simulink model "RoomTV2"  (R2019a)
settings: Solver=ode15s  StartTime=0.0  StopTime=tend  RelTol=1e-3
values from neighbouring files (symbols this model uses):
  ACmax = 4.5    [mainV3.m]    (also in mainV3_SRC.m)
  ACmin = 0    [mainV3.m]    (also in mainV3_SRC.m)
  EHmax = 4    [mainV3.m]    (also in mainV3_SRC.m)
  EHmin = 0    [mainV3.m]    (also in mainV3_SRC.m)
  HWmax = 3    [mainV3.m]    (also in mainV3_SRC.m)
  HWmin = 0    [mainV3.m]    (also in mainV3_SRC.m)
  Kc_ac = tau_ac/(K_ac*(tauc_ac+theta_ac))    (= -1.23666666667)    [RoomTuning.m]
  Kc_eh = tau_eh/(K_eh*(tauc_eh+theta_eh))    (= 1.23666666667)    [RoomTuning.m]
  Kc_hw = tau_hw/(K_hw*(tauc_hw+theta_hw))    (= 3.13641025641)    [RoomTuning.m]
  KI_ac = Kc_ac/tauI_ac    [RoomTuning.m]
  KI_eh = Kc_eh/tauI_eh    [RoomTuning.m]
  KI_hw = Kc_hw/tauI_hw    [RoomTuning.m]
  m_in0 = 0.4    [mainOL.m]    (also in mainV3.m; mainV3_SRC.m)
  p = [m,Cp, Ufl, Afl, mfl, Cpfl]'    [mainOL.m]    (also in mainV3.m; mainV3_SRC.m)
  par_ac = [p_ac, m_in0, Cp, kT]'    [mainV3.m]    (also in mainV3_SRC.m)
  par_el = [p_el, m_in0, Cp, kT]'    [mainV3.m]    (also in mainV3_SRC.m)
  par_hw = [p_hw, m_in0, Cp, kT]'    [mainV3.m]    (also in mainV3_SRC.m)
  par_J = [p_el, p_hw, p_ac, m_in0, kv, kT]'    [mainV3.m]    (also in mainV3_SRC.m)
  QAC0 = 0    [mainOL.m]    (also in mainV3.m; mainV3_SRC.m)
  QH10 = 0    [mainOL.m]    (also in mainV3.m; mainV3_SRC.m)
  QH20 = 0    [mainOL.m]    (also in mainV3.m; mainV3_SRC.m)
  Tdes0 = T0    (= 21)    [mainV3.m]    (also in mainV3_SRC.m)
  x0 = [T0; Tfl0]    [mainOL.m]    (also in mainV3.m; mainV3_SRC.m; col_obj.m = 0.5*ones(1,82)'; Simulate1Col.m = x)
undefined symbols (not defined in the file or in its folder): objRoom, Room, spQac, spQel, spQhw
libraries: simulink x3

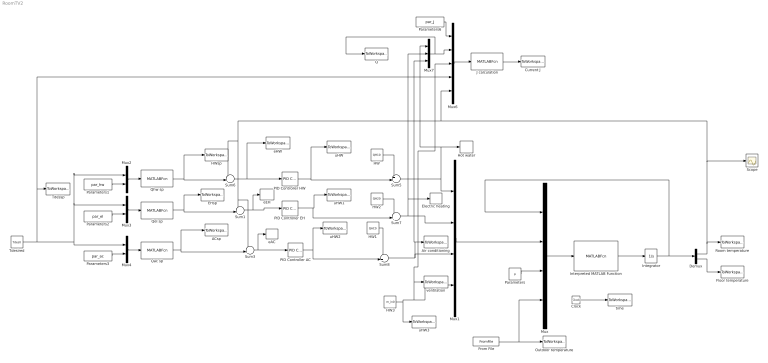
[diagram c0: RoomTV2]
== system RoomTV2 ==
  ACsp : ToWorkspace  VariableName=ACsp  SampleTime=-1
  Air conditioning : ToWorkspace  VariableName=QAC  SampleTime=-1
  Clock : Clock
  Current J : ToWorkspace  VariableName=Jactual  SampleTime=-1
  Demux : Demux  Outputs=2
  EHsp : ToWorkspace  VariableName=EHsp  SampleTime=-1
  Electric heating : ToWorkspace  VariableName=QH2  SampleTime=-1
  Floor temperature : ToWorkspace  VariableName=Tfl  SampleTime=-1
  From File : FromFile  FileName=Tambient.mat  OutDataTypeStr=double  SampleTime=0
  HW : Constant  Value=QH10
  HW1 : Constant  Value=QAC0
  HW2 : Constant  Value=QH20
  HW3 : Constant  Value=m_in0
  HWsp : ToWorkspace  VariableName=HWsp  SampleTime=-1
  Hot water : ToWorkspace  VariableName=QH1  SampleTime=-1
  Integrator : Integrator  InitialCondition=x0'
  Interpreted MATLAB Function : MATLABFcn  MATLABFcn=Room(u)  OutputDimensions=2  Output1D=off
  J calculation : MATLABFcn  MATLABFcn=objRoom(u)  OutputDimensions=1  Output1D=off
  Mux : Mux
  Mux1 : Mux
  Mux2 : Mux  Inputs=2
  Mux3 : Mux  Inputs=2
  Mux4 : Mux  Inputs=2
  Mux6 : Mux  Inputs=5
  Mux7 : Mux  Inputs=3
  Outdoor temperature : ToWorkspace  VariableName=Tin  SampleTime=-1
  PID Controller AC : simulink/Continuous/PID Controller  Controller=PI  Form=Parallel  TimeDomain=Continuous-time  SampleTime=-1  IntegratorMethod=Forward Euler  FilterMethod=Forward Euler  ControllerParametersSource=internal  P=Kc_ac  I=KI_ac  D=0  UseFilter=on  N=100  TunerSelectOption=Transfer Function Based (PID Tuner App)  InitialConditionSource=internal  InitialConditionForIntegrator=0  InitialConditionForFilter=0  DifferentiatorICPrevScaledInput=0  ExternalReset=none  TrackingMode=off  Kt=1  LimitOutput=on  UpperSaturationLimit=ACmax  LowerSaturationLimit=ACmin  LinearizeAsGain=on  AntiWindupMode=back-calculation  Kb=1  POutMin=[]  POutMax=[]  IOutMin=[]  IOutMax=[]  DOutMin=[]  DOutMax=[]  NOutMin=[]  NOutMax=[]  SumOutMin=[]  SumOutMax=[]  SaturationOutMin=[]  SaturationOutMax=[]  PParamMin=[]  PParamMax=[]  IParamMin=[]  IParamMax=[]  DParamMin=[]  DParamMax=[]  NParamMin=[]  NParamMax=[]  KbParamMin=[]  KbParamMax=[]  KtParamMin=[]  KtParamMax=[]  KbOutMin=[]  KbOutMax=[]  KtOutMin=[]  KtOutMax=[]  IntegratorOutMin=[]  IntegratorOutMax=[]  FilterOutMin=[]  FilterOutMax=[]  SumI1OutMin=[]  SumI1OutMax=[]  SumI2OutMin=[]  SumI2OutMax=[]  SumI3OutMin=[]  SumI3OutMax=[]  SumI4OutMin=[]  SumI4OutMax=[]  SumDOutMin=[]  SumDOutMax=[]  DifferentiatorOutMin=[]  DifferentiatorOutMax=[]  FilterDiffOutCoefMin=[]  FilterDiffOutCoefMax=[]  ReciprocalOutMin=[]  ReciprocalOutMax=[]  SumDenOutMin=[]  SumDenOutMax=[]  SumNumOutMin=[]  SumNumOutMax=[]  DivideOutMin=[]  DivideOutMax=[]  IntegratorContinuousStateAttributes=''  IntegratorStateMustResolveToSignalObject=off  IntegratorRTWStateStorageClass=Auto  FilterContinuousStateAttributes=''  FilterStateMustResolveToSignalObject=off  FilterRTWStateStorageClass=Auto  ParallelPVariant=InternalParameters  IdealPVariant=Disabled  IVariant=InternalParameters  DVariant=Disabled  IntegratorVariant=Continuous  SatVariant=Enabled  AWVariant=BackCalculation  PCopyVariant=Disabled  TRVariant=Disabled  FdbkBlocksVariant=Forward  IdealPFdbkVariant=Disabled  SatFdbkVariant=Disabled  DerivativeFilterVariant=Disabled  NVariant=Disabled  NCopyVariant=Disabled_SignalSpec  FilterICVariant=Disabled  IntegratorICVariant=InternalICs  ExternalResetVariant=Disabled  TRSumVariant=Passthrough  SumFdbkVariant=Disabled  SumVariant=Sum_PI
  PID Controller EH : simulink/Continuous/PID Controller  Controller=PI  Form=Parallel  TimeDomain=Continuous-time  SampleTime=-1  IntegratorMethod=Forward Euler  FilterMethod=Forward Euler  ControllerParametersSource=internal  P=Kc_eh  I=KI_eh  D=0  UseFilter=on  N=100  TunerSelectOption=Transfer Function Based (PID Tuner App)  InitialConditionSource=internal  InitialConditionForIntegrator=0  InitialConditionForFilter=0  DifferentiatorICPrevScaledInput=0  ExternalReset=none  TrackingMode=off  Kt=1  LimitOutput=on  UpperSaturationLimit=EHmax  LowerSaturationLimit=EHmin  LinearizeAsGain=on  AntiWindupMode=clamping  Kb=1  POutMin=[]  POutMax=[]  IOutMin=[]  IOutMax=[]  DOutMin=[]  DOutMax=[]  NOutMin=[]  NOutMax=[]  SumOutMin=[]  SumOutMax=[]  SaturationOutMin=[]  SaturationOutMax=[]  PParamMin=[]  PParamMax=[]  IParamMin=[]  IParamMax=[]  DParamMin=[]  DParamMax=[]  NParamMin=[]  NParamMax=[]  KbParamMin=[]  KbParamMax=[]  KtParamMin=[]  KtParamMax=[]  KbOutMin=[]  KbOutMax=[]  KtOutMin=[]  KtOutMax=[]  IntegratorOutMin=[]  IntegratorOutMax=[]  FilterOutMin=[]  FilterOutMax=[]  SumI1OutMin=[]  SumI1OutMax=[]  SumI2OutMin=[]  SumI2OutMax=[]  SumI3OutMin=[]  SumI3OutMax=[]  SumI4OutMin=[]  SumI4OutMax=[]  SumDOutMin=[]  SumDOutMax=[]  DifferentiatorOutMin=[]  DifferentiatorOutMax=[]  FilterDiffOutCoefMin=[]  FilterDiffOutCoefMax=[]  ReciprocalOutMin=[]  ReciprocalOutMax=[]  SumDenOutMin=[]  SumDenOutMax=[]  SumNumOutMin=[]  SumNumOutMax=[]  DivideOutMin=[]  DivideOutMax=[]  IntegratorContinuousStateAttributes=''  IntegratorStateMustResolveToSignalObject=off  IntegratorRTWStateStorageClass=Auto  FilterContinuousStateAttributes=''  FilterStateMustResolveToSignalObject=off  FilterRTWStateStorageClass=Auto  ParallelPVariant=InternalParameters  IdealPVariant=Disabled  IVariant=InternalParameters  DVariant=Disabled  IntegratorVariant=Continuous  SatVariant=Enabled  AWVariant=ContClampingParallel  PCopyVariant=Disabled  TRVariant=Disabled  FdbkBlocksVariant=Forward  IdealPFdbkVariant=Disabled  SatFdbkVariant=Disabled  DerivativeFilterVariant=Disabled  NVariant=Disabled  NCopyVariant=Disabled_SignalSpec  FilterICVariant=Disabled  IntegratorICVariant=InternalICs  ExternalResetVariant=Disabled  TRSumVariant=Passthrough  SumFdbkVariant=Disabled  SumVariant=Sum_PI
  PID Controller HW : simulink/Continuous/PID Controller  Controller=PI  Form=Parallel  TimeDomain=Continuous-time  SampleTime=-1  IntegratorMethod=Forward Euler  FilterMethod=Forward Euler  ControllerParametersSource=internal  P=Kc_hw  I=KI_hw  D=0  UseFilter=on  N=100  TunerSelectOption=Transfer Function Based (PID Tuner App)  InitialConditionSource=internal  InitialConditionForIntegrator=0  InitialConditionForFilter=0  DifferentiatorICPrevScaledInput=0  ExternalReset=none  TrackingMode=off  Kt=1  LimitOutput=on  UpperSaturationLimit=HWmax  LowerSaturationLimit=HWmin  LinearizeAsGain=on  AntiWindupMode=clamping  Kb=1  POutMin=[]  POutMax=[]  IOutMin=[]  IOutMax=[]  DOutMin=[]  DOutMax=[]  NOutMin=[]  NOutMax=[]  SumOutMin=[]  SumOutMax=[]  SaturationOutMin=[]  SaturationOutMax=[]  PParamMin=[]  PParamMax=[]  IParamMin=[]  IParamMax=[]  DParamMin=[]  DParamMax=[]  NParamMin=[]  NParamMax=[]  KbParamMin=[]  KbParamMax=[]  KtParamMin=[]  KtParamMax=[]  KbOutMin=[]  KbOutMax=[]  KtOutMin=[]  KtOutMax=[]  IntegratorOutMin=[]  IntegratorOutMax=[]  FilterOutMin=[]  FilterOutMax=[]  SumI1OutMin=[]  SumI1OutMax=[]  SumI2OutMin=[]  SumI2OutMax=[]  SumI3OutMin=[]  SumI3OutMax=[]  SumI4OutMin=[]  SumI4OutMax=[]  SumDOutMin=[]  SumDOutMax=[]  DifferentiatorOutMin=[]  DifferentiatorOutMax=[]  FilterDiffOutCoefMin=[]  FilterDiffOutCoefMax=[]  ReciprocalOutMin=[]  ReciprocalOutMax=[]  SumDenOutMin=[]  SumDenOutMax=[]  SumNumOutMin=[]  SumNumOutMax=[]  DivideOutMin=[]  DivideOutMax=[]  IntegratorContinuousStateAttributes=''  IntegratorStateMustResolveToSignalObject=off  IntegratorRTWStateStorageClass=Auto  FilterContinuousStateAttributes=''  FilterStateMustResolveToSignalObject=off  FilterRTWStateStorageClass=Auto  ParallelPVariant=InternalParameters  IdealPVariant=Disabled  IVariant=InternalParameters  DVariant=Disabled  IntegratorVariant=Continuous  SatVariant=Enabled  AWVariant=ContClampingParallel  PCopyVariant=Disabled  TRVariant=Disabled  FdbkBlocksVariant=Forward  IdealPFdbkVariant=Disabled  SatFdbkVariant=Disabled  DerivativeFilterVariant=Disabled  NVariant=Disabled  NCopyVariant=Disabled_SignalSpec  FilterICVariant=Disabled  IntegratorICVariant=InternalICs  ExternalResetVariant=Disabled  TRSumVariant=Passthrough  SumFdbkVariant=Disabled  SumVariant=Sum_PI
  Parameters : Constant  Value=p
  Parameters1 : Constant  Value=par_hw
  Parameters2 : Constant  Value=par_el
  Parameters3 : Constant  Value=par_ac
  Parameters6 : Constant  Value=par_J
  Q : ToWorkspace  VariableName=Q  SampleTime=-1
  Qac sp : MATLABFcn  MATLABFcn=spQac(u)  OutputDimensions=1  Output1D=off
  Qel sp : MATLABFcn  MATLABFcn=spQel(u)  OutputDimensions=1  Output1D=off
  Qhw sp : MATLABFcn  MATLABFcn=spQhw(u)  OutputDimensions=1  Output1D=off
  Room temperature : ToWorkspace  VariableName=T  SampleTime=-1
  Scope : Scope
  Sum1 : Sum  Inputs=-+|
  Sum3 : Sum  Inputs=-+|
  Sum5 : Sum  Inputs=++|
  Sum6 : Sum  Inputs=-+|
  Sum7 : Sum  Inputs=++|
  Sum8 : Sum  Inputs=++|
  Tdesired : Constant  Value=Tdes0
  Tdessp : ToWorkspace  VariableName=Tdes_sp  SampleTime=-1
  eAC : ToWorkspace  VariableName=eAC  SampleTime=-1
  eEH : ToWorkspace  VariableName=eEH  SampleTime=-1
  eHW : ToWorkspace  VariableName=eHW  SampleTime=-1
  time : ToWorkspace  VariableName=t  SampleTime=-1
  uHW : ToWorkspace  VariableName=uHW  SampleTime=-1
  uHW1 : ToWorkspace  VariableName=uEH  SampleTime=-1
  uHW2 : ToWorkspace  VariableName=uAC  SampleTime=-1
  uHW3 : ToWorkspace  VariableName=u_mv  SampleTime=-1
  ventilation : ToWorkspace  VariableName=m_in  SampleTime=-1
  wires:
  Clock/1 -> time/1
  Interpreted MATLAB Function/1 -> Integrator/1
  Mux/1 -> Interpreted MATLAB Function/1
  Integrator/1 -> Demux/1, Mux/1
  Parameters/1 -> Mux/3
  Mux1/1 -> Mux/2
  Demux/1 -> Mux6/5, Sum6/1, Sum3/1, Sum1/1, Scope/1, Room temperature/1
  Demux/2 -> Floor temperature/1
  Tdesired/1 -> Mux6/4, Tdessp/1, Mux3/1, Mux2/1, Mux4/1
  Qhw sp/1 -> Sum6/2, HWsp/1
  Mux2/1 -> Qhw sp/1
  Mux3/1 -> Qel sp/1
  Mux4/1 -> Qac sp/1
  Parameters1/1 -> Mux2/2
  Parameters2/1 -> Mux3/2
  Parameters3/1 -> Mux4/2
  Qel sp/1 -> EHsp/1, Sum1/2
  Qac sp/1 -> ACsp/1, Sum3/2
  Sum3/1 -> eAC/1, PID Controller AC/1
  Sum6/1 -> eHW/1, PID Controller HW/1
  PID Controller HW/1 -> uHW/1, Sum5/2
  Sum1/1 -> eEH/1, PID Controller EH/1
  PID Controller EH/1 -> Sum7/2, uHW1/1
  PID Controller AC/1 -> uHW2/1, Sum8/2
  Sum5/1 -> Mux1/1, Mux7/1, Hot water/1
  HW/1 -> Sum5/1
  Sum7/1 -> Mux7/2, Electric heating/1, Mux1/2
  HW2/1 -> Sum7/1
  Sum8/1 -> Mux7/3, Air conditioning/1, Mux1/3
  HW1/1 -> Sum8/1
  J calculation/1 -> Current J/1
  Mux6/1 -> J calculation/1
  HW3/1 -> Mux6/3, ventilation/1, Mux1/4, uHW3/1
  Parameters6/1 -> Mux6/1
  Mux7/1 -> Q/1, Mux6/2
  From File/1 -> Outdoor temperature/1, Mux/4
